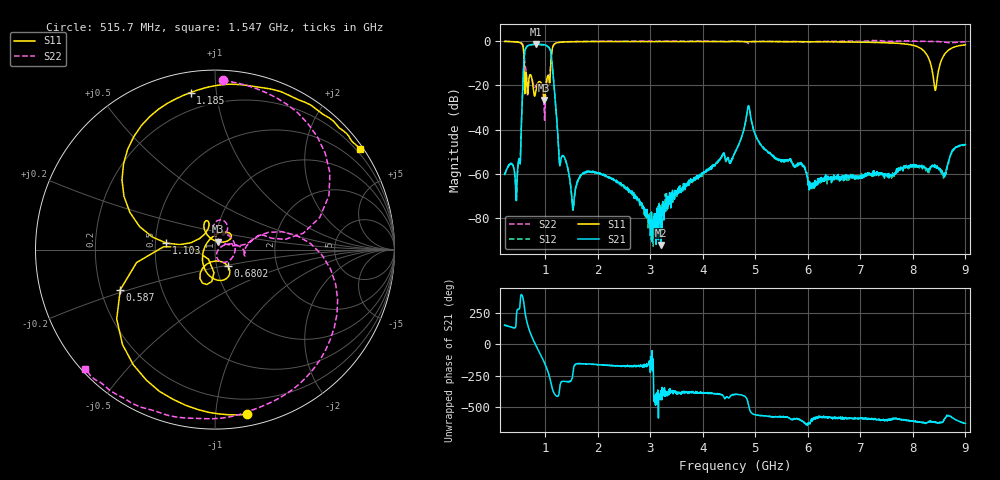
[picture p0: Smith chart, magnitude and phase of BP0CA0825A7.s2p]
!Agilent Technologies,E8358A,US41080443,A.07.50.56
!Agilent E8358A: A.07.50.56
!Date: Thursday, November 09, 2017 08:53:15
!Correction: S11(Full 2 Port(1,2))
!S21(Full 2 Port(1,2))
!S12(Full 2 Port(1,2))
!S22(Full 2 Port(1,2))
!S2P File: Measurements: S11, S21, S12, S22:
# Hz S  dB  R 50
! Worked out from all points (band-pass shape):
!   1601 points, 225 MHz to 9 GHz, reference 50 ohm
!   highest |S21| = -1.28 dB at 822.8 MHz (marker M1); lowest = -92.2 dB at 3.198 GHz (marker M2)
!   |S21| within 3 dB of the highest: 611.8 MHz to 1.098 GHz (486.1 MHz wide, 56.9 % of centre)
!   lowest |S11| = -26.6 dB at 981.8 MHz (marker M3), VSWR 1.10, Z = 51.4 + j4.56 ohm
!   |S11| at or under -10 dB: 596.7 MHz to 1.105 GHz (508.8 MHz wide, 59.8 % of centre); 8.336 GHz to 8.522 GHz (185.9 MHz wide, 2.21 % of centre)
!   |S22| runs from -35.7 to 0.4 dB; largest |S21 - S12| = 0.016
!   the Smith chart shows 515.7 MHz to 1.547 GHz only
!   S11 on the Smith chart (normalised r, x): 515.7 MHz: 0.08, -1.21; 587 MHz: 0.28, -0.19; 680.2 MHz: 1.13, -0.21; 1.103 GHz: 0.57, +0.05; 1.185 GHz: 0.10, +0.85; 1.547 GHz: 0.11, +3.19
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2.25e8  -0.08 -19.7  -60.28 152.1  -60.24 152.3  -0.03 153.5
4.44375e8  -0.28 -53.7  -71.76 178.7  -71.48 176.7  -0.24 113.1
5.156719e8  -0.58 -79.1  -54.75 -58.3  -54.92 -57.4  -0.50 87.3
5.869688e8  -4.84 -157.1  -11.75 -18.1  -11.93 -17.8  -3.07 25.4
6.802031e8  -18.72 -52.1  -1.83 132.3  -1.99 132.5  -19.57 94.0
8.227969e8  -22.19 93.4  -1.28 -10.8  -1.43 -10.6  -20.10 61.7
9.050625e8  -18.36 41.6  -1.36 -78.7  -1.52 -78.5  -19.23 -14.1
9.818438e8  -26.55 70.5  -1.57 -145.8  -1.72 -145.7  -33.74 -59.7
1.1025e9  -11.23 172.4  -4.77 59.6  -4.94 59.8  -10.05 17.9
1.184766e9  -1.05 98.9  -25.31 -42.8  -25.42 -42.7  -1.08 -57.5
1.278e9  -0.42 68.1  -56.09 22.7  -56.43 21.4  -0.49 -95.3
1.546734e9  -0.17 34.8  -72.02 -176.5  -71.49 -173.2  -0.14 -137.6
1.689328e9  -0.18 25.6  -60.22 -155.6  -60.47 -155.0  -0.09 -149.1
3.153656e9  -0.15 -22.3  -89.85 130.1  -79.82 -76.6  0.07 -176.6
3.197531e9  -0.17 -23.8  -92.16 -11.6  -75.66 -46.6  0.03 -176.6
4.6125e9  -0.08 -48.8  -50.35 -40.6  -50.30 -40.9  0.02 168.3
4.87575e9  -0.18 -52.2  -29.28 -137.8  -29.48 -138.0  -0.94 166.0
6.076828e9  -0.22 -72.3  -66.30 105.9  -65.39 116.6  -0.27 142.3
7.541156e9  -0.74 -121.7  -59.79 117.8  -59.92 116.7  -0.06 115.6
8.325422e9  -9.21 146.9  -57.97 101.4  -57.35 103.5  -0.11 105.2
8.429625e9  -22.25 37.9  -56.94 98.1  -56.87 95.5  -0.09 103.5
9e9  -1.57 -129.0  -46.72 86.4  -46.99 86.9  -0.23 100.3
